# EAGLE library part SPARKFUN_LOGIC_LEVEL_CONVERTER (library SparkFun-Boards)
SparkFun Logic Level Converter -Bi-Directional This is the mechnical outline for the 3.3V - 5V bi directional logic level converter. SparkFun Products: SparkFun Logic Level Converter - Bi-Directional
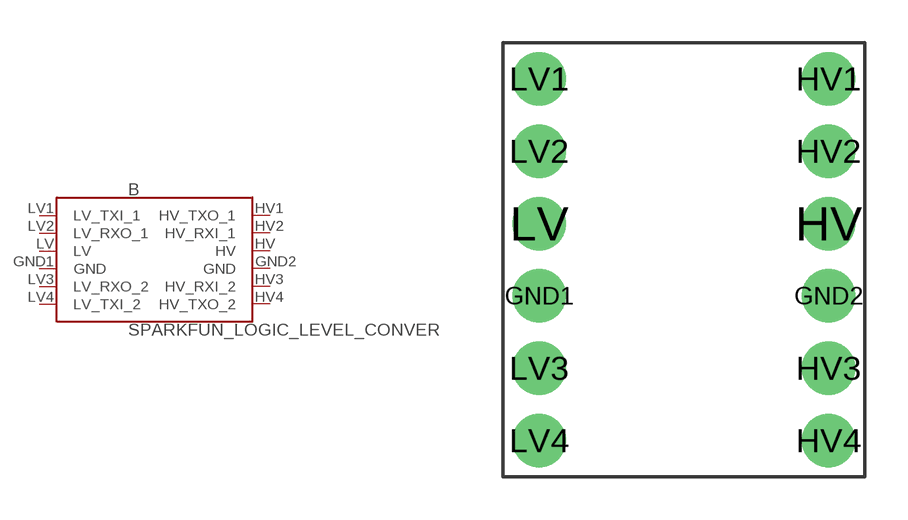
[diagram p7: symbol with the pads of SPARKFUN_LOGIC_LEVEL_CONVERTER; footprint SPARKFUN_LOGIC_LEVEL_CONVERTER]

Designator prefix B

## SPARKFUN_LOGIC_LEVEL_CONVERTER  [SPARKFUN_LOGIC_LEVEL_CONVERTER]
GND1  GND  pwr
GND2  GND  pwr
HV  HV  pwr
HV1  HV_TXO_1
HV2  HV_RXI_1
HV3  HV_RXI_2
HV4  HV_TXO_2
LV  LV  pwr
LV1  LV_TXI_1
LV2  LV_RXO_1
LV3  LV_RXO_2
LV4  LV_TXI_2

## Footprint SPARKFUN_LOGIC_LEVEL_CONVERTER (pad centres in mm)
SparkFun Logic Level Converter Specifications: Pin count:12 Pin pitch: 0.1" Area: 0.6x 0.5 " Example device(s): SparkFun Logic Level Converter
drill 1.016 pad 1.88: GND1 -5.08,-1.27; GND2 5.08,-1.27; HV 5.08,1.27; HV1 5.08,6.35; HV2 5.08,3.81; HV3 5.08,-3.81; HV4 5.08,-6.35; LV -5.08,1.27; LV1 -5.08,6.35; LV2 -5.08,3.81; LV3 -5.08,-3.81; LV4 -5.08,-6.35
